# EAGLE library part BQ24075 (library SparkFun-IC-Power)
Texas Instruments BQ24075 LiPo Battery Chargerand Power-Path Management IC The bq2407x series of devices are integrated Li-Ion linear chargers and system power path management devices targeted at space-limited portable applications. The devices operate from either a USB port or an AC adapter and support charge currents up to 1.5 A. The input voltage range with input overvoltage protection supports unregulated adapters. The USB input current limit accuracy and start up sequence allow the bq2407x to meet USB-IF inrush current specifications. Additionally, the input dynamic power management (VIN-DPM) prevents the charger from crashing incorrectly configured USB sources. Datasheet SparkFun Products SparkFun Battery Babysitter (PRT-13777)
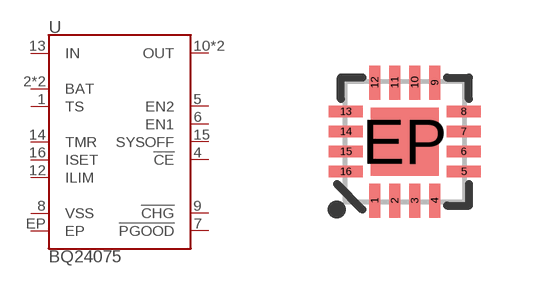
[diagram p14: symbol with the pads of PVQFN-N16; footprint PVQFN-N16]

Designator prefix U

## BQ24075 (PROD_ID: IC-13219)  [PVQFN-N16]
1  TS
2  BAT
3  BAT
4  !CE!
5  EN2
6  EN1
7  !PGOOD!
8  VSS
9  !CHG!
10  OUT
11  OUT
12  ILIM
13  IN
14  TMR
15  SYSOFF
16  ISET
EP  EP

## Footprint PVQFN-N16 (pad centres in mm)
16-Pin VSON (VQFN) 3.0 x 3.0 mm IC Dimensions: 3.0 x3.0 x 1.0 mm Pitch: 0.5mm Pins: 16 + Bottom Pad Used by the BQ24075 LiPo Charger Example Datasheet
smd 0.28 x 0.85: 1 -0.75,-1.475; 2 -0.25,-1.475; 3 0.25,-1.475; 4 0.75,-1.475; 9 0.75,1.475; 10 0.25,1.475; 11 -0.25,1.475; 12 -0.75,1.475
smd 0.85 x 0.28: 5 1.475,-0.75; 6 1.475,-0.25; 7 1.475,0.25; 8 1.475,0.75; 13 -1.475,0.75; 14 -1.475,0.25; 15 -1.475,-0.25; 16 -1.475,-0.75
smd 1.7 x 1.7: EP 0,0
